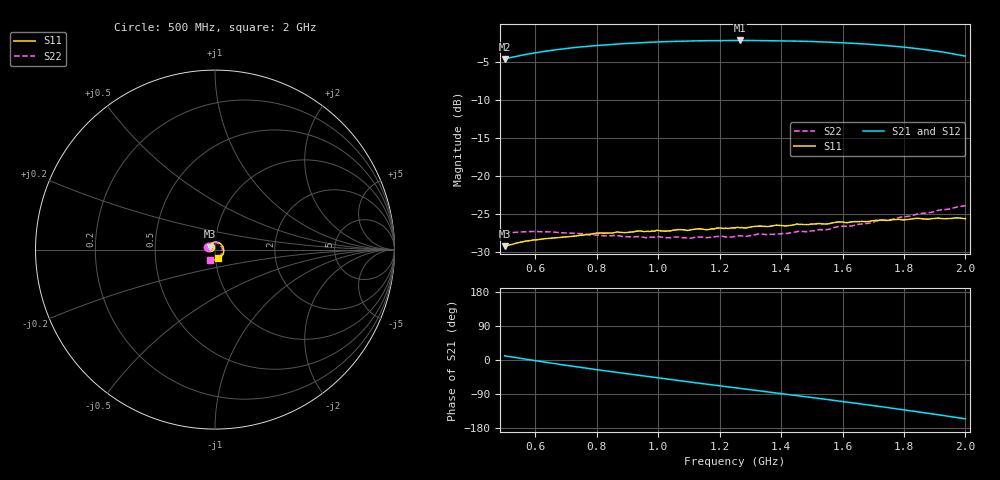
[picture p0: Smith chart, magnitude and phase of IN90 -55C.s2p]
!Agilent Technologies,E8363B,SG43030131,A.07.50.48
!Agilent E8363B: A.07.50.48
!Date: Friday, October 17, 2025 03:53:49
!Correction: S11(Full 2 Port(1,2))
!S21(Full 2 Port(1,2))
!S12(Full 2 Port(1,2))
!S22(Full 2 Port(1,2))
!S2P File: Measurements: S11, S21, S12, S22:
# Hz S  dB  R 50
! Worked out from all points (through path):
!   201 points, 500 MHz to 2 GHz, reference 50 ohm
!   highest |S21| = -2.20 dB at 1.265 GHz (marker M1); lowest = -4.6 dB at 500 MHz (marker M2)
!   lowest |S11| = -29.3 dB at 500 MHz (marker M3), VSWR 1.07, Z = 47.1 + j1.58 ohm
!   |S11| at or under -10 dB: start of sweep to end of sweep
!   |S22| runs from -28.3 to -23.9 dB; largest |S21 - S12| = 0.0015
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5e8  -29.27 150.9  -4.64 11.0  -4.63 11.0  -27.58 159.7
5.6e8  -28.68 136.9  -4.12 3.2  -4.11 3.2  -27.38 146.6
6.2e8  -28.35 125.0  -3.69 -4.3  -3.69 -4.3  -27.37 134.5
6.8e8  -28.13 113.9  -3.36 -11.6  -3.36 -11.6  -27.48 122.9
7.55e8  -27.84 100.4  -3.03 -20.4  -3.03 -20.4  -27.64 107.6
8.75e8  -27.45 82.3  -2.65 -33.8  -2.65 -33.8  -27.90 83.5
9.575e8  -27.35 70.7  -2.47 -42.7  -2.47 -42.8  -28.15 67.0
1.0025e9  -27.22 64.5  -2.39 -47.6  -2.40 -47.5  -28.01 58.7
1.1e9  -27.17 52.0  -2.27 -57.8  -2.28 -57.8  -28.25 40.2
1.1225e9  -27.02 49.0  -2.26 -60.1  -2.25 -60.1  -28.06 36.1
1.25e9  -26.87 33.4  -2.20 -73.2  -2.20 -73.3  -27.98 13.2
1.265e9  -26.85 30.8  -2.20 -74.8  -2.20 -74.8  -27.90 9.8
1.3925e9  -26.53 16.0  -2.24 -87.9  -2.24 -87.9  -27.66 -12.4
1.505e9  -26.36 3.6  -2.35 -99.5  -2.35 -99.5  -27.26 -31.3
1.5575e9  -26.30 -2.9  -2.43 -105.0  -2.42 -105.0  -27.04 -41.2
1.5875e9  -26.07 -7.2  -2.48 -108.2  -2.48 -108.2  -26.67 -46.1
1.6325e9  -26.06 -11.9  -2.57 -113.0  -2.56 -113.0  -26.58 -53.1
1.7525e9  -25.86 -28.1  -2.91 -126.1  -2.90 -126.2  -25.81 -73.9
1.8425e9  -25.60 -42.4  -3.27 -136.3  -3.27 -136.4  -25.05 -88.4
1.88e9  -25.71 -48.0  -3.46 -140.8  -3.46 -140.7  -24.88 -95.1
1.9325e9  -25.67 -57.8  -3.76 -147.0  -3.77 -146.9  -24.47 -104.7
2e9  -25.65 -71.4  -4.26 -155.3  -4.25 -155.2  -23.93 -116.5
